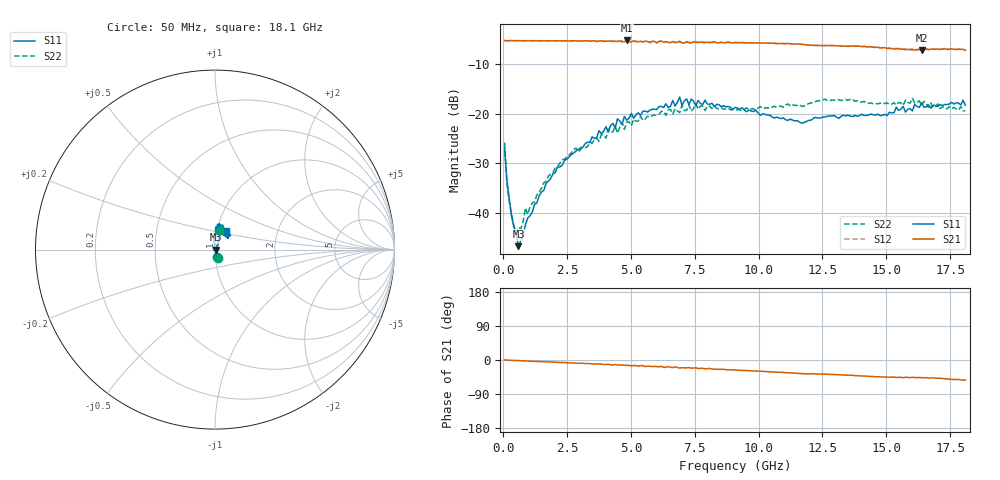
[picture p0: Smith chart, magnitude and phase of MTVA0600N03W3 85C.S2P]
! Network Analyzer HP8720D.06.14 Serial No. US36140669
!  8 Jul 2005  10:11:59
! Frequency  S11  S21  S12  S22
# HZ  S  DB R 50
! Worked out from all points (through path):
!   201 points, 50 MHz to 18.1 GHz, reference 50 ohm
!   highest |S21| = -5.19 dB at 4.833 GHz (marker M1); lowest = -7.2 dB at 16.39 GHz (marker M2)
!   group delay of S21, straight-line fit = 8.16 ps
!   lowest |S11| = -46.7 dB at 591.5 MHz (marker M3), VSWR 1.01, Z = 50.5 - j0.0484 ohm
!   |S11| at or under -10 dB: start of sweep to end of sweep
!   |S22| runs from -44.0 to -16.9 dB; largest |S21 - S12| = 0.021
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5e7  -27.05 -75.4  -5.20 0.0  -5.22 0.3  -25.83 -72.9
1.4025e8  -33.48 -68.4  -5.28 -0.3  -5.25 -0.3  -34.11 -98.8
2.305e8  -37.11 -60.9  -5.23 -0.6  -5.22 -0.6  -37.68 -113.7
5.0125e8  -44.39 -24.2  -5.25 -1.5  -5.23 -1.5  -43.96 -165.9
5.915e8  -46.74 -6.0  -5.22 -1.5  -5.25 -1.5  -42.91 176.6
6.8175e8  -45.66 12.5  -5.24 -1.9  -5.25 -2.0  -43.24 162.8
8.6225e8  -42.47 35.0  -5.24 -2.3  -5.25 -2.4  -39.03 150.6
9.525e8  -41.08 41.9  -5.25 -2.5  -5.23 -2.7  -40.33 135.0
1.6745e9  -34.01 56.5  -5.25 -4.8  -5.25 -4.8  -33.66 106.0
3.1185e9  -26.70 67.9  -5.28 -8.7  -5.31 -9.1  -26.69 99.2
4.021e9  -22.59 70.4  -5.32 -11.9  -5.35 -11.3  -24.92 92.2
4.11125e9  -23.72 69.8  -5.30 -11.2  -5.33 -12.3  -23.08 91.7
4.47225e9  -21.01 66.7  -5.39 -13.1  -5.29 -12.4  -23.91 95.7
4.83325e9  -21.30 76.6  -5.19 -13.8  -5.32 -14.6  -21.71 84.0
6.09675e9  -18.55 74.4  -5.40 -17.8  -5.32 -17.8  -20.14 84.1
6.909e9  -16.63 80.4  -5.35 -21.1  -5.47 -20.0  -19.76 77.8
7.54075e9  -18.36 77.6  -5.55 -20.6  -5.42 -22.7  -17.96 83.8
9.075e9  -18.71 86.6  -5.61 -26.4  -5.59 -26.5  -19.13 75.5
1.21435e10  -20.92 72.1  -6.16 -36.4  -6.12 -36.6  -17.73 73.9
1.512175e10  -19.71 44.5  -6.82 -45.7  -6.69 -45.4  -18.09 75.8
1.638525e10  -17.80 51.0  -7.15 -46.6  -6.99 -46.2  -18.34 72.4
1.81e10  -18.27 60.5  -7.15 -52.6  -7.27 -53.5  -19.38 75.5
